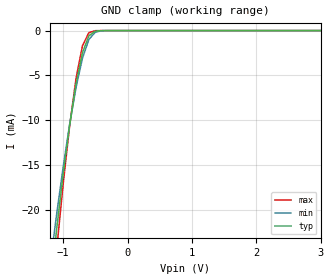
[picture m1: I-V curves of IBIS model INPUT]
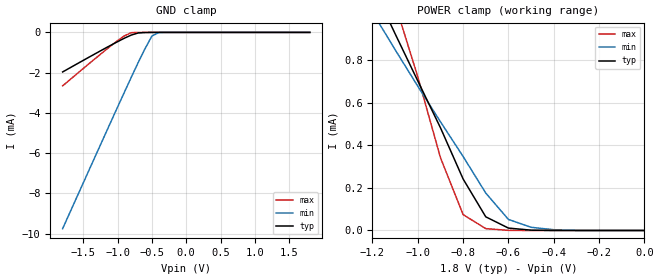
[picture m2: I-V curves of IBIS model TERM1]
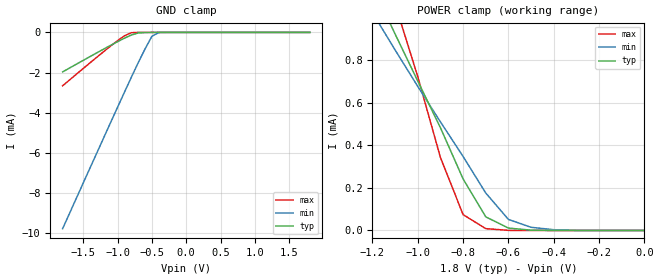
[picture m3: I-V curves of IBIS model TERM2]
|   PERICOM SEMICONDUCTOR CORP
|   IBIS Model of PI3A223
|   Product Family: 3A
|   UQFN-10 (ZM) Package
[IBIS Ver] 3.2
[Comment char] |_char
[File Name] pi3a223_zm_18v.ibs
[File Rev] 1.0
[Source] File originated at Pericom Semiconductor Corp.
[Date] 08/14/17
[Disclaimer] (C) Copyright PERICOM Semiconductor Corporation
   All rights reserved
  Pericom Semiconductor Corporation hereby grants the user of
  this IBIS model a non-exclusive, nontransferable license to
  use this IBIS model under the following terms.
  This IBIS model is provided on an "AS IS" basis and Pericom
  makes absolutely no warranty with respect to the information
  contained herein. PERICOM DISCLAIMS AND CUSTOMER WAIVES ALL
  WARRANTIES, EXPRESSED OR IMPLIED, INCLUDING WARRANTIES OF
  MERCHANTABILITY OR FITNESS FOR A PARTICULAR PURPOSE. The
  entire risk as to quality and performance is with the customer.
  Accordingly, in no event shall the company be liable for any
  damages, whether in contract or tort, including any lost
  profits or other incidental, consequential, exemplary, or
  punitive damages arising out of the use or application of the
  IBIS model provided in this package. Further, Pericom reserves
  the right to make changes without notice to any product herein
  to improve reliability, function, or design. Pericom does not
  convey any license under patent rights or any other intellectual
  property rights, including those of third parties.
  The user is granted this license only to use the IBIS model
  and is not granted rights to sell, load, rent, lease or license
  the IBIS model in whole or in part, or in modified form to anyone
  other than user. User may modify the IBIS model to suit its specific
  application but rights to derivative works and such modifications
  shall belong to Pericom.
  Pericom is not obligated to provide maintenance or support
  for the licensed IBIS model.
  Contact Pericom at ATTN: APPLICATION ENGINEERING / IBIS MODELS
  2380 Bering Drive, San Jose, CA 95131
[Component] PI3A223
[Manufacturer] Pericom Semiconductor Corp.
[Package]
| variable   typ   min   max
R_pkg   0.10120ohm   0.09060ohm   0.11180ohm
L_pkg   1.24800nH   1.01600nH   1.48000nH
C_pkg   0.22300pF   0.20300pF   0.24400pF
[Pin] signal_name   model_name   R_pin   L_pin   C_pin
1   VDD   POWER   0.10120   1.24800nH   0.22300pF
2   NO1   TERM1   0.10120   1.24800nH   0.22300pF
3   COM1   TERM2   0.11180   1.48000nH   0.24400pF
4   IN1   INPUT   0.09060   1.01600nH   0.20200pF
5   NC1   TERM1   0.11180   1.48000nH   0.24400pF
6   GND   GND   0.10120   1.24800nH   0.22300pF
7   NC2   TERM1   0.10120   1.24800nH   0.22300pF
8   IN2   INPUT   0.11180   1.48000nH   0.24400pF
9   COM2   TERM2   0.09060   1.01600nH   0.20200pF
10   NO2   TERM1   0.11180   1.48000nH   0.24400pF
[Series Switch Groups]
On 1 /
Off 2 /
[Series Pin Mapping]   pin_2   model_name  function_table_group
5   3   SWITCH1   1
2   3   SWITCH1   2
7   9   SWITCH1   1
10   9   SWITCH1   2
|   Model SWITCH1
[Model] SWITCH1
Model_type Series_switch
| variable   typ   min   max
C_comp   69.00pF   68.70pF   69.30pF
[Voltage Range]   1.8000V   1.6200V   1.9800V
[GND Clamp Reference]   0.0000V   0.0000V   0.0000V
[POWER Clamp Reference]   1.8000V   1.6200V   1.9800V
[Temperature Range]   25   85   -40
[On]
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[OFF]
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| Models and submodels in the file (4): INPUT (Input), SWITCH1 (Series_switch), TERM1 (Terminator), TERM2 (Terminator)
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|   Model INPUT
[Model] INPUT
Model_type Input
Vinl = 420mV
Vinh = 1.36V
| variable   typ   min   max
C_comp   0.950pF   0.940pF   0.960pF
[Voltage Range]   1.8000V   1.6200V   1.9800V
[GND Clamp Reference]   0.0000V   0.0000V   0.0000V
[POWER Clamp Reference]   1.8000V   1.6200V   1.9800V
[Temperature Range]   25   85   -40
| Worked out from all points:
|   GND clamp passes 1 mA (typ) near -0.62 V on its own axis
[GND Clamp]
| Voltage   I(typ)   I(min)   I(max)
-1.8V     -72.02mA   -63.61mA   -82.57mA
-1.2V     -28.62mA   -26.02mA   -32.15mA
-1.1V     -22.12mA   -20.45mA   -24.4mA
-1V       -16.06mA   -15.24mA   -17.17mA
-900mV    -10.6mA    -10.51mA   -10.7mA
-800mV    -5.96mA    -6.37mA    -5.35mA
-700mV    -2.471mA   -3.08mA    -1.693mA
-600mV    -576.6uA   -991.2uA   -224.1uA
-500mV    -63.68uA   -177.5uA   -11.66uA
-400mV    -4.071uA   -19.39uA   -284nA
3.6V      90.57pA    920.9pA    72.05pA
[POWER Clamp]   |Note: Vtable = Vcc - Voutput
| Voltage   I(typ)   I(min)   I(max)
-1.8V     0A         0A         0A
0V        0A         0A         0A
|   Model TERM1
[Model] TERM1
Model_type Terminator
| variable   typ   min   max
C_comp   28.00pF   27.90pF   28.10pF
[Voltage Range]   1.8000V   1.6200V   1.9800V
[GND Clamp Reference]   0.0000V   0.0000V   0.0000V
[POWER Clamp Reference]   1.8000V   1.6200V   1.9800V
[Temperature Range]   25   85   -40
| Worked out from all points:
|   GND clamp passes 1 mA (typ) near -1.29 V on its own axis
|   POWER clamp passes 1 mA (typ) near -1.13 V on its own axis
[GND Clamp]
| Voltage   I(typ)   I(min)   I(max)
-1.8V     -1.966mA   -9.756mA   -2.657mA
-1.2V     -826.1uA   -5.218mA   -950.2uA
-900mV    -288uA     -2.968mA   -169.2uA
-800mV    -132.1uA   -2.227mA   -15.8uA
-700mV    -28.5uA    -1.5mA     -150.3nA
-600mV    -6.527uA   -810.8uA   -4.157nA
-500mV    -1.251uA   -181.6uA   -1.231nA
-400mV    -27.66nA   -7.773uA   -798.9pA
1.8V      193.3pA    7.511nA    152.6pA
[POWER Clamp]   |Note: Vtable = Vcc - Voutput
| Voltage   I(typ)   I(min)   I(max)
-1.8V     2.591mA    2.153mA    3.506mA
-1.2V     1.149mA    1.024mA    1.398mA
-1.1V     923.1uA    848.5uA    1.063mA
-1V       701.9uA    677uA      721.7uA
-900mV    482.3uA    510.3uA    342.1uA
-800mV    241.8uA    347.3uA    74.49uA
-700mV    64.03uA    175.6uA    8.645uA
-600mV    11.24uA    51.87uA    507.2nA
-500mV    1.456uA    14.94uA    15.61nA
-400mV    61.14nA    3.55uA     877.4pA
0V        1.944nA    330.5pA    11.75nA
|   Model TERM2
[Model] TERM2
Model_type Terminator
| variable   typ   min   max
C_comp   41.0pF   40.8pF   41.2pF
[Voltage Range]   1.8000V   1.6200V   1.9800V
[GND Clamp Reference]   0.0000V   0.0000V   0.0000V
[POWER Clamp Reference]   1.8000V   1.6200V   1.9800V
[Temperature Range]   25   85   -40
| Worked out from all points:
|   GND clamp passes 1 mA (typ) near -1.29 V on its own axis
|   POWER clamp passes 1 mA (typ) near -1.13 V on its own axis
[GND Clamp]
| Voltage   I(typ)   I(min)   I(max)
-1.8V     -1.967mA   -9.772mA   -2.658mA
-1.2V     -826.4uA   -5.231mA   -950.6uA
-900mV    -288.2uA   -2.98mA    -169.3uA
-800mV    -132.2uA   -2.239mA   -15.8uA
-700mV    -28.52uA   -1.513mA   -150.3nA
-500mV    -1.253uA   -192.5uA   -1.23nA
-400mV    -27.66nA   -7.919uA   -798.4pA
1.8V      316.5pA    7.515nA    265.2pA
[POWER Clamp]   |Note: Vtable = Vcc - Voutput
| Voltage   I(typ)   I(min)   I(max)
-1.8V     2.593mA    2.154mA    3.508mA
-1.2V     1.15mA     1.025mA    1.399mA
-1.1V     923.9uA    849.1uA    1.065mA
-1V       702.8uA    677.7uA    723.4uA
-900mV    483.3uA    510.9uA    343.2uA
-800mV    242.5uA    348uA      74.62uA
-700mV    64.16uA    176.1uA    8.646uA
-600mV    11.24uA    52uA       507.3nA
-500mV    1.456uA    14.95uA    15.62nA
-400mV    61.14nA    3.551uA    889.3pA
0V        316.5pA    344.3pA    338pA
